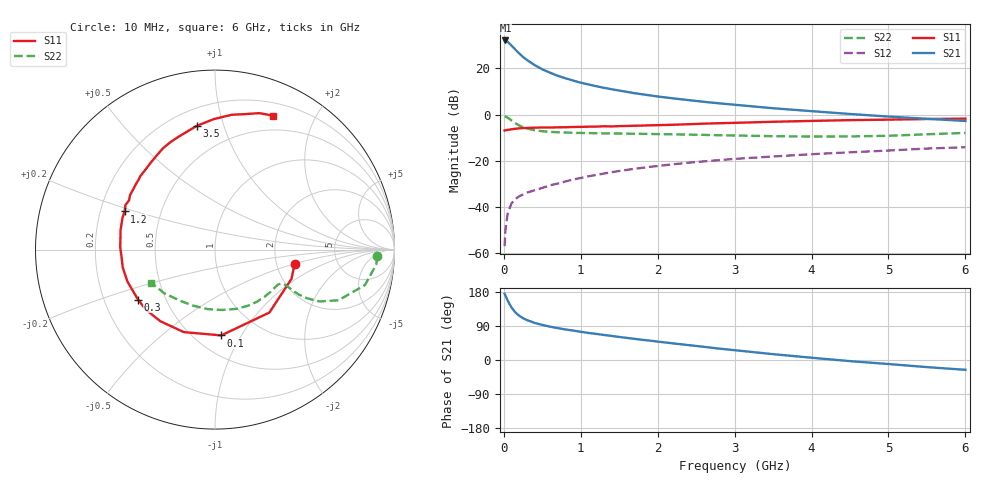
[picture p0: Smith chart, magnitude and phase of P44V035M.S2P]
! SIEMENS Small Signal Semiconductors
! BFP182
! Si NPN RF Bipolar Junction Transistor in SOT143
! VCE = 4 V  IC = 35 mA
! Common Emitter S-Parameters:  March  1996
# GHz  S  MA  R  50
!  f  S11  S21  S12  S22
! GHz  MAG  ANG  MAG  ANG  MAG  ANG  MAG  ANG
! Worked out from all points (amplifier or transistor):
!   36 points, 10 MHz to 6 GHz, reference 50 ohm
!   highest |S21| = 32.1 dB at 20 MHz (marker M1)
!   |S21| within 3 dB of that: start of sweep to 122.3 MHz
!   unconditionally stable (mu >= 1): start of sweep to 12.88 MHz; 410.8 MHz to end of sweep
!   at 250 MHz: K = 0.75, MSG = 29.8 dB, |S12| = -34.7 dB
!   at 1.4 GHz: K = 1.37, MAG = 14.4 dB, |S12| = -25.0 dB
!   at 6 GHz: K = 1.01, MAG = 5.1 dB, |S12| = -14.2 dB
!   S11 on the Smith chart (normalised r, x): 10 MHz: 2.53, -0.50; 100 MHz: 0.66, -0.82; 300 MHz: 0.35, -0.26; 1.2 GHz: 0.30, +0.18; 3.5 GHz: 0.30, +0.81; 6 GHz: 0.33, +1.47
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0.01  0.4508 -10.0  40.3 174.9  0.0014 74.2  0.906 -2.3
0.02  0.4563 -21.0  40.37 170.4  0.0031 82.9  0.9022 -5.3
0.05  0.4634 -49.2  37.87 156.6  0.0072 74.0  0.8584 -13.3
0.1  0.4793 -85.8  31.24 138.5  0.0119 58.8  0.7441 -22.3
0.15  0.4914 -110.7  25.58 125.6  0.0148 52.8  0.6497 -26.4
0.2  0.5019 -127.3  21.08 116.7  0.0169 51.5  0.5788 -27.9
0.25  0.5101 -138.9  17.68 110.2  0.0184 51.5  0.5304 -28.2
0.3  0.5115 -147.0  15.26 105.5  0.0202 51.1  0.4984 -27.9
0.4  0.5192 -159.9  11.81 97.9  0.0228 52.9  0.4573 -27.0
0.5  0.5235 -169.1  9.54 92.5  0.0257 53.6  0.4349 -26.7
0.6  0.5225 -176.0  8.097 88.0  0.0292 55.2  0.4215 -26.8
0.7  0.5284 178.4  6.924 84.1  0.0318 56.7  0.4127 -27.4
0.8  0.5305 173.3  6.123 80.6  0.0354 57.9  0.407 -28.2
1.1  0.5451 161.0  4.486 71.4  0.0458 58.6  0.3959 -31.7
1.2  0.5469 157.1  4.115 68.9  0.049 58.6  0.3935 -33.1
1.7  0.5717 140.7  2.9 55.8  0.0666 56.9  0.3828 -41.5
2.2  0.6004 127.2  2.242 43.8  0.0834 53.5  0.3727 -51.3
2.8  0.648 112.6  1.749 30.0  0.1027 48.0  0.3555 -64.9
3.5  0.6965 98.5  1.37 15.4  0.1232 41.8  0.3389 -83.1
4.5  0.7567 83.0  1.028 -3.0  0.1519 32.9  0.3355 -111.9
5.5  0.7994 72.0  0.81 -18.8  0.1831 24.2  0.3732 -139.5
6  0.8135 66.5  0.725 -25.9  0.1955 18.8  0.3996 -152.4
